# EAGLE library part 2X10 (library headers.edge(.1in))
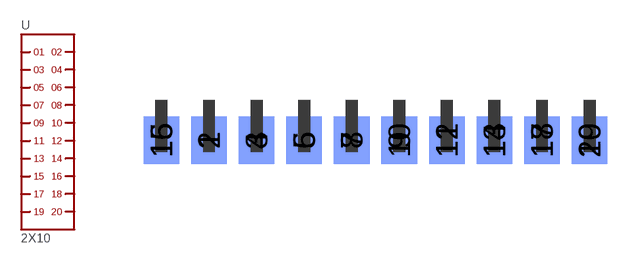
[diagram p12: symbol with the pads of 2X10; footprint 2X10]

Designator prefix -

## 2X10  [2X10]
1  1
2  2
3  3
4  4
5  5
6  6
7  7
8  8
9  9
10  10
11  11
12  12
13  13
14  14
15  15
16  16
17  17
18  18
19  19
20  20

## Footprint 2X10 (pad centres in mm)
smd 1.905 x 2.54: 1 2.54,-2.159; 3 5.08,-2.159; 5 7.62,-2.159; 7 10.16,-2.159; 9 12.7,-2.159; 11 15.24,-2.159; 13 17.78,-2.159; 15 0,-2.159; 17 20.32,-2.159; 19 22.86,-2.159
smd 1.905 x 2.54 bottom: 2 2.54,-2.159; 4 5.08,-2.159; 6 7.62,-2.159; 8 10.16,-2.159; 10 12.7,-2.159; 12 15.24,-2.159; 14 17.78,-2.159; 16 0,-2.159; 18 20.32,-2.159; 20 22.86,-2.159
